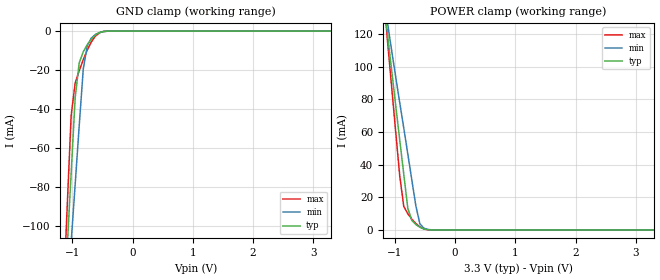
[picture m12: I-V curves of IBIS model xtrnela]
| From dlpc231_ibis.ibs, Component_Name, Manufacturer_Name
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[Model] xtrnela
Model_type Input
Polarity   Non-Inverting
Enable   Active-High
Vinl =  0.800V
Vinh =  2.000V
C_comp   1.467pF   1.337pF   1.607pF
C_comp_pullup   0.739pF   0.729pF   0.858pF
C_comp_pulldown   0.739pF   0.729pF   0.858pF
[Temperature Range]   25.000   0.125k   -40.000
[Voltage Range]   3.300V   2.970V   3.630V
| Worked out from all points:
|   GND clamp passes 1 mA (typ) near -0.56 V on its own axis
|   POWER clamp passes 1 mA (typ) near -0.54 V on its own axis
[GND_clamp]
|Voltage   I(typ)   I(min)   I(max)
-3.3V     -1.427A    -1.15A     -1.714A
-1.156V   -150.4mA   -167.4mA   -139.2mA
-1.089V   -111.5mA   -137.6mA   -90.81mA
-1.022V   -72.74mA   -108mA     -43.25mA
-955mV    -34.03mA   -78.35mA   -26.51mA
-888mV    -16.28mA   -48.39mA   -20.26mA
-821mV    -10.62mA   -19.49mA   -14.65mA
-754mV    -6.923mA   -7.441mA   -9.664mA
-687mV    -4.068mA   -3.577mA   -5.579mA
-620mV    -2.019mA   -1.775mA   -2.607mA
-419mV    -41.36uA   -61.09uA   -33.17uA
3.3V      0A         0A         0A
[POWER_clamp]
|Voltage   I(typ)   I(min)   I(max)
-3.3V     1.021A     835.1mA    1.212A
-1.189V   141.3mA    142.8mA    142.9mA
-1.122V   119.4mA    126.3mA    115mA
-1.055V   97.69mA    109.9mA    87.42mA
-921mV    55.11mA    77.95mA    33.12mA
-854mV    34.13mA    62.46mA    14.45mA
-787mV    13.31mA    46.58mA    9.94mA
-720mV    5.843mA    30.55mA    6.638mA
-653mV    3.311mA    14.71mA    3.922mA
-586mV    1.672mA    3.755mA    1.886mA
-385mV    21.64uA    65.49uA    10.69uA
3.3V      0A         0A         0A
